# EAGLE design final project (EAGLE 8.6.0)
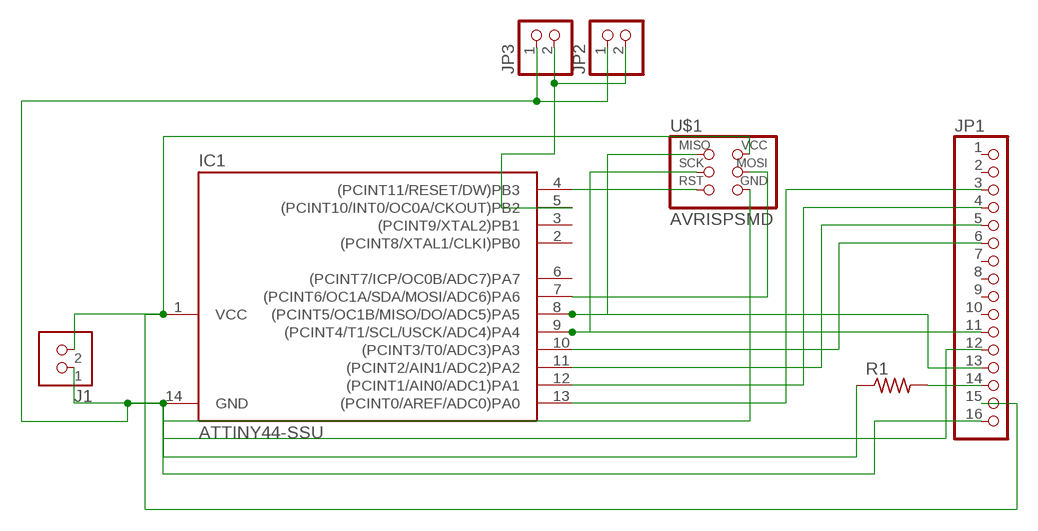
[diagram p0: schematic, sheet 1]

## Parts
IC1  ATTINY44-SSU  [SOIC14]
J1  TERM-1X02-FABLAB  [ED555DS-2DS]
JP1  PINHD-1X16  [1X16]
JP2  PINHD-1X2  [1X02]
JP3  PINHD-1X2  [1X02]
R1  RES-US1206FAB  [R1206FAB]
U$1  AVRISPSMD  [2X03SMD]

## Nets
N$1: IC1.4((PCINT11/RESET/DW)PB3) U$1.5(RST)
N$2: IC1.9((PCINT4/T1/SCL/USCK/ADC4)PA4) JP1.11 U$1.3(SCK)
N$3: IC1.8((PCINT5/OC1B/MISO/DO/ADC5)PA5) JP1.13 U$1.1(MISO)
N$4: IC1.7((PCINT6/OC1A/SDA/MOSI/ADC6)PA6) U$1.4(MOSI)
N$5: IC1.5((PCINT10/INT0/OC0A/CKOUT)PB2) JP2.2 JP3.2
N$6: IC1.1(VCC) J1.2 JP1.15 U$1.2(VCC)
N$7: IC1.13((PCINT0/AREF/ADC0)PA0) JP1.3
N$8: IC1.12((PCINT1/AIN0/ADC1)PA1) JP1.4
N$9: IC1.11((PCINT2/AIN1/ADC2)PA2) JP1.5
N$10: IC1.10((PCINT3/T0/ADC3)PA3) JP1.6
N$11: JP1.14 R1.2
N$12: IC1.14(GND) J1.1 JP1.12 JP1.16 JP2.1 JP3.1 R1.1 U$1.6(GND)
Unconnected: IC1.2((PCINT8/XTAL1/CLKI)PB0) IC1.3((PCINT9/XTAL2)PB1) IC1.6((PCINT7/ICP/OC0B/ADC7)PA7) JP1.1 JP1.2 JP1.7 JP1.8 JP1.9 JP1.10

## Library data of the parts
IC1 = fab:ATTINY44
J1 = fab:TERM-1X02: 3.5mm terminal block, 2 positions ED555-2DS as found in the fablab inventory.
JP1 = pinhead:PINHD-1X16: PIN HEADER
JP2 JP3 = pinhead:PINHD-1X2: PIN HEADER
R1 = fab:RES-US: Resistor (US Symbol)
U$1 = fab:AVRISP

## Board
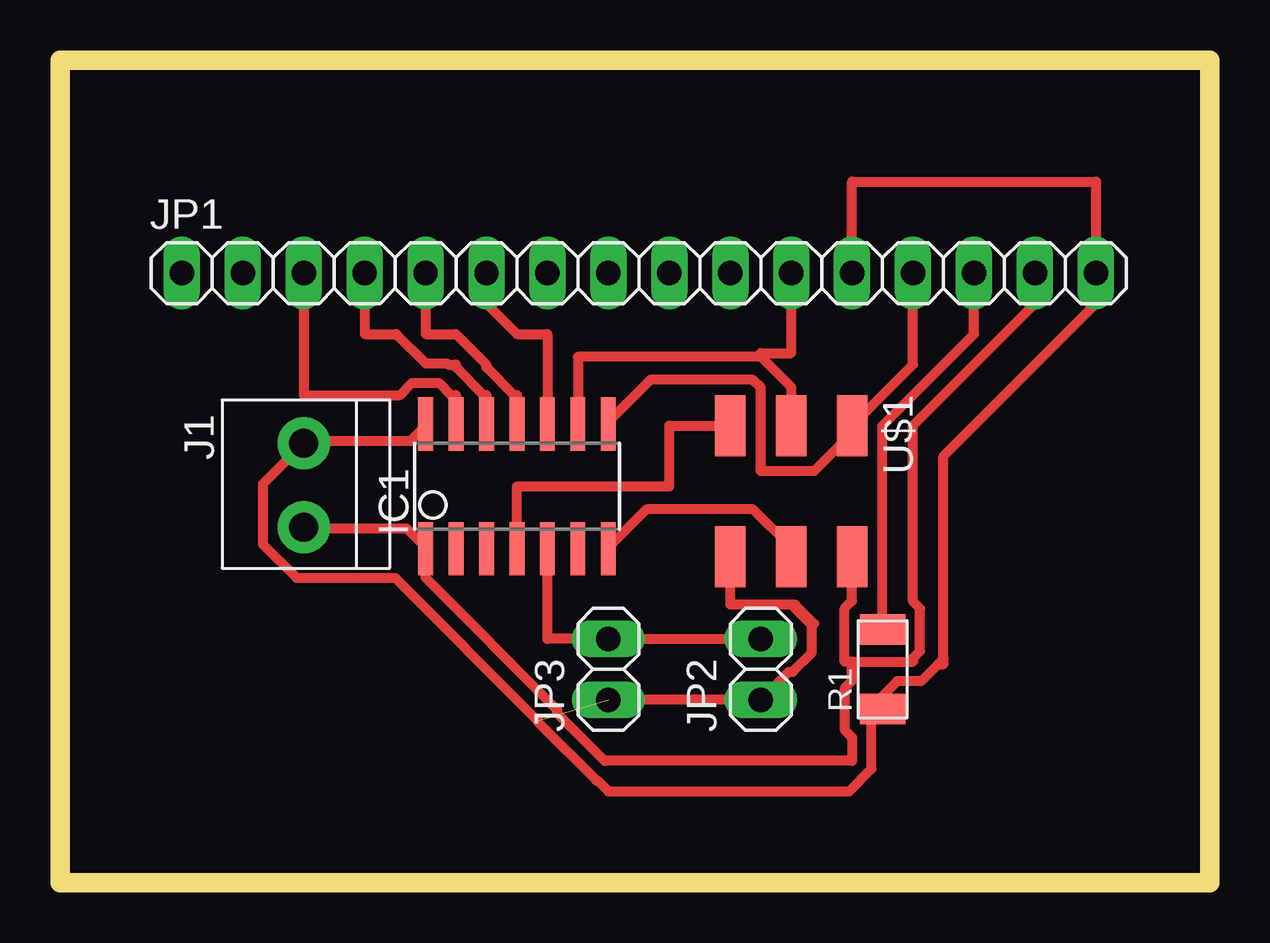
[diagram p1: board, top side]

Size 47.93 x 34.28 mm. Coordinates in mm from the lower left corner, seen from the top.
Outline: 0,0 47.93,0 47.93,34.28 0,34.28 0,0
Copper layers (1*16): Top 0.035mm / dielectric 1.5mm / Bottom 0.035mm
Design rules "default *": minimum track width 16mil, minimum drill 0.35mm, track to track 16mil, track to pad 16mil, pad to pad 16mil, via to via 16mil, smd to smd 16mil, copper to edge 16mil, drill to drill 16mil, minimum pad ring 10mil, minimum via ring 8mil, stop-mask expansion 4mil, vias tented up to drill 0mil, thermal gap 10mil

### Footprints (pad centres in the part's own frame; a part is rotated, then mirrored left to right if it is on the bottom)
SOIC14 = smd 0.61 x 2.21: 1 -3.81,-2.603; 2 -2.54,-2.603; 3 -1.27,-2.603; 4 0,-2.603; 5 1.27,-2.603; 6 2.54,-2.603; 7 3.81,-2.603; 8 3.81,2.603; 9 2.54,2.603; 10 1.27,2.603; 11 0,2.603; 12 -1.27,2.603; 13 -2.54,2.603; 14 -3.81,2.603
ED555DS-2DS = drill 1.2 pad 2.184: 1 1.8,0; 2 -1.7,0
1X16 = drill 1.016 long: 1 -19.05,0; 2 -16.51,0; 3 -13.97,0; 4 -11.43,0; 5 -8.89,0; 6 -6.35,0; 7 -3.81,0; 8 -1.27,0; 9 1.27,0; 10 3.81,0; 11 6.35,0; 12 8.89,0; 13 11.43,0; 14 13.97,0; 15 16.51,0; 16 19.05,0
1X02 = drill 1.016 long: 1 -1.27,0; 2 1.27,0
R1206FAB = smd 1.27 x 1.905: 1 -1.651,0; 2 1.651,0
2X03SMD = smd 2.54 x 1.27: 1 -2.54,2.54; 2 2.92,2.54; 3 -2.54,0; 4 2.92,0; 5 -2.54,-2.54; 6 2.92,-2.54

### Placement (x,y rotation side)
IC1  19.05,16.51 0 top
J1  10.16,16.51 90 top
JP1  24.13,25.4 0 top
JP2  29.21,8.89 90 top
JP3  22.86,8.89 90 top
R1  34.29,8.89 90 top
U$1  30.48,16.51 270 top

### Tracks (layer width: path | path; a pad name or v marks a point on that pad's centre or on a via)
N$1
  Top 0.406: IC1.4 19.05,16.51 25.4,16.51 25.4,19.05 U$1.5
N$2
  Top 0.406: IC1.9 21.59,21.91 29.21,21.91 | 29.21,21.91 30.48,20.64 U$1.3 | JP1.11 30.48,22.07 29.21,22.07 29.21,21.91
N$3
  Top 0.406: U$1.1 33.02,18.73 31.43,17.15 29.21,17.15 29.21,20.64 28.89,20.95 24.61,20.95 22.86,19.21 IC1.8 | 33.02,19.21 U$1.1 | U$1.1 35.56,21.59 JP1.13
N$4
  Top 0.406: U$1.4 30.48,13.97 28.89,15.56 24.45,15.56 22.86,13.97 IC1.7
N$5
  Top 0.406: IC1.5 20.32,10.16 JP3.2 JP2.2
N$6
  Top 0.406: J1.2 10.16,14.76 14.45,14.76 15.24,13.97 IC1.1 15.24,12.7 20.73,7.21 20.73,7.05 22.7,5.08 33.02,5.08 33.02,6.06 32.73,6.35 32.73,8.13 33.02,8.42 33.02,9.21 | U$1.2 33.02,11.75 32.7,11.43 32.7,9.21 33.02,9.21 | 33.02,9.21 35.56,9.21 35.56,9.36 35.85,9.65 35.85,11.43 35.56,11.72 35.56,19.05 40.64,24.13 JP1.15
N$7
  Top 0.406: 10.16,25.08 JP1.3 10.16,20.32 14.18,20.32 14.68,20.83 15.8,20.83 16.3,20.32 16.51,20.32 IC1.13
N$8
  Top 0.406: 12.7,25.08 JP1.4 12.7,22.86 14.02,22.86 15.24,21.64 16.13,21.64 16.19,21.59 16.51,21.59 16.51,21.47 17.66,20.32 17.78,20.32 IC1.12
N$9
  Top 0.406: 15.24,25.08 JP1.5 15.24,22.86 16.51,22.86 17.78,21.59 17.78,21.47 18.93,20.32 19.05,20.32 IC1.11
N$10
  Top 0.406: JP1.6 17.78,24.13 19.05,22.86 20.32,22.86 IC1.10
N$11
  Top 0.406: 38.26,25.4 JP1.14 38.1,22.86 34.29,19.05 R1.2 34.29,10.64
N$12  (1 unrouted)
  Top 0.406: JP1.16 43.18,25.72 | IC1.14 15.24,19.05 14.61,18.41 10.16,18.41 J1.1 8.46,16.61 8.46,14.11 9.86,12.7 13.97,12.7 19.91,6.76 19.91,6.72 22.36,4.27 22.4,4.27 22.86,3.81 32.9,3.81 33.83,4.74 33.83,6.84 34.29,7.3 | 33.97,7.62 34.29,7.3 | 34.29,7.3 R1.1 34.29,7.78 34.91,8.4 35.9,8.4 36.61,9.11 | U$1.6 27.94,11.59 30.64,11.59 | 31.43,10.8 30.64,11.59 | 22.86,7.78 JP3.1 JP2.1 30.38,8.79 30.54,8.79 31.34,9.59 31.34,10.73 30.64,11.43 30.64,11.59 | 36.61,9.11 36.83,9.33 | JP1.16 43.18,24.13 36.83,17.78 36.83,9.11 36.61,9.11 | JP1.12 33.02,29.21 43.18,29.21 JP1.16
